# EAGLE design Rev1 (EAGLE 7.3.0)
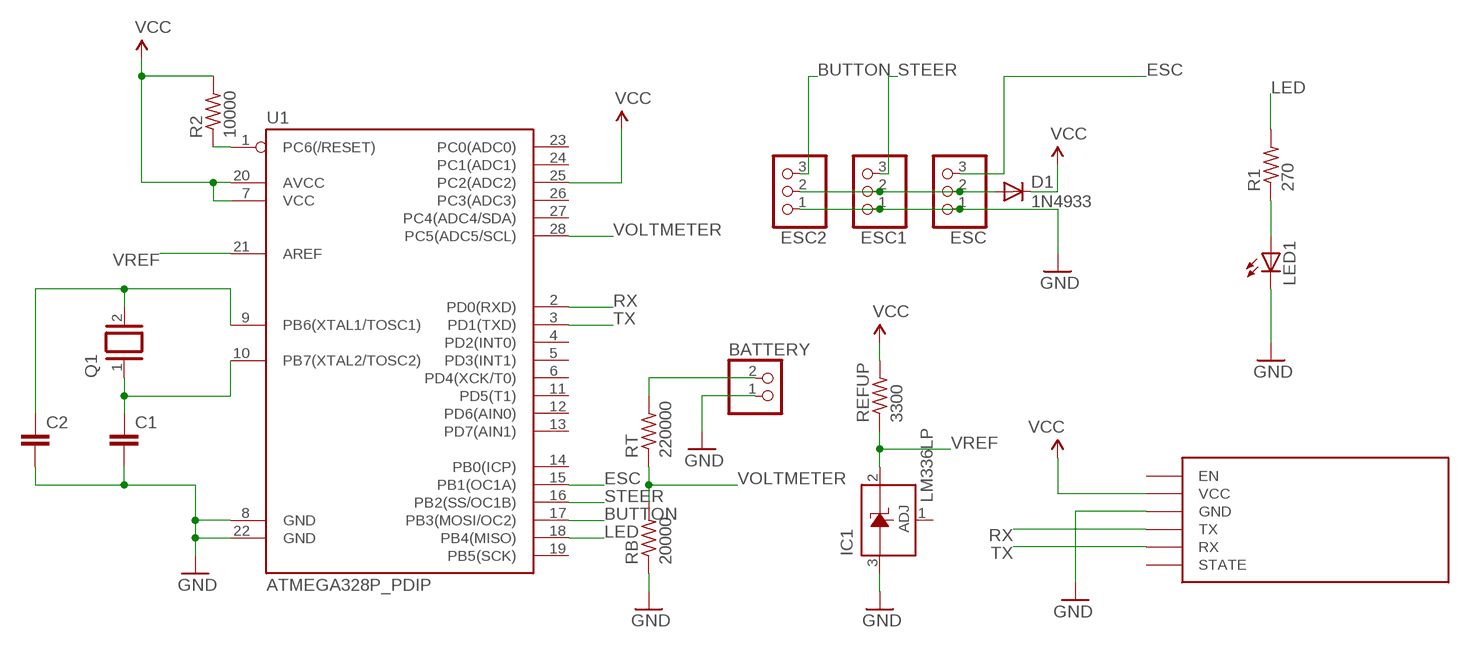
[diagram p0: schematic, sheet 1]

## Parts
BATTERY  JST_2PIN-THM  [JST-PH-2-THM]
C1  C2.5/4  [C2.5-4]
C2  C2.5/4  [C2.5-4]
D1  1N4933  [DO41-10]
ESC  PINHD-1X3  [1X03]
ESC1  PINHD-1X3  [1X03]
ESC2  PINHD-1X3  [1X03]
IC1  LM336LP  [TO92]
LED1  LED5MM  [LED5MM]
Q1  XTAL/S  [QS]
R1  270  R-US_0204/7  [0204/7]
R2  10000  R-US_0207/7  [0207/7]
RB  20000  R-US_0204/7  [0204/7]
REFUP  3300  R-US_0204/7  [0204/7]
RT  220000  R-US_0204/7  [0204/7]
U1  ATMEGA328P_PDIP  [DIL28-3]
U$1  HC06  [HC06]

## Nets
BUTTON: ESC2.3 U1.17(PB3(MOSI/OC2))
ESC: ESC.3 U1.15(PB1(OC1A))
GND: BATTERY.1 C1.2 C2.2 ESC1.1 ESC2.1 ESC.1 IC1.3(A) LED1.K(C) RB.1 U1.8(GND) U1.22(GND) U$1.GND
LED: R1.2 U1.18(PB4(MISO))
N$2: LED1.A R1.1
N$3: C1.1 Q1.1 U1.10(PB7(XTAL2/TOSC2))
N$4: BATTERY.2 RT.2
N$5: C2.1 Q1.2 U1.9(PB6(XTAL1/TOSC1))
N$7: R2.1 U1.1(PC6(/RESET))
N$10: D1.A ESC1.2 ESC2.2 ESC.2
RX: U1.2(PD0(RXD)) U$1.TX
STEER: ESC1.3 U1.16(PB2(SS/OC1B))
TX: U1.3(PD1(TXD)) U$1.RX
VCC: D1.C R2.2 REFUP.2 U1.7(VCC) U1.20(AVCC) U1.25(PC2(ADC2)) U$1.VCC
VOLTMETER: RB.2 RT.1 U1.28(PC5(ADC5/SCL))
VREF: IC1.2(C) REFUP.1 U1.21(AREF)
Unconnected: IC1.1(ADJ) U1.4(PD2(INT0)) U1.5(PD3(INT1)) U1.6(PD4(XCK/T0)) U1.11(PD5(T1)) U1.12(PD6(AIN0)) U1.13(PD7(AIN1)) U1.14(PB0(ICP)) U1.19(PB5(SCK)) U1.23(PC0(ADC0)) U1.24(PC1(ADC1)) U1.26(PC3(ADC3)) U1.27(PC4(ADC4/SDA)) U$1.EN U$1.STATE

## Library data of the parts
BATTERY = adafruit:JST_2PIN: JST 2-Pin Connectors of various flavors
C1 C2 = capacitor-wima:C: CAPACITOR
D1 = diode:1N4933: DIODE
ESC ESC1 ESC2 = pinhead:PINHD-1X3: PIN HEADER
IC1 = VLADLIBRARY:LM336: 2.5-V INTEGRATED REFERENCE CIRCUITS LM236 Source: http://focus.ti.com/lit/ds/symlink/lm336-2.5.pdf
LED1 = adafruit:LED: LED
Q1 = special:XTAL/S: CRYSTAL
R1 RB REFUP RT = adafruit:R-US_: RESISTOR, American symbol
R2 = resistor:R-US_: RESISTOR, American symbol
U1 = SparkFun-DigitalIC:ATMEGA328P_PDIP: uC used in the Arduino 32kb flash, 1k EEPROM, 2k SRAM This is the through-hole version of this chip.
U$1 = ccs:HC06

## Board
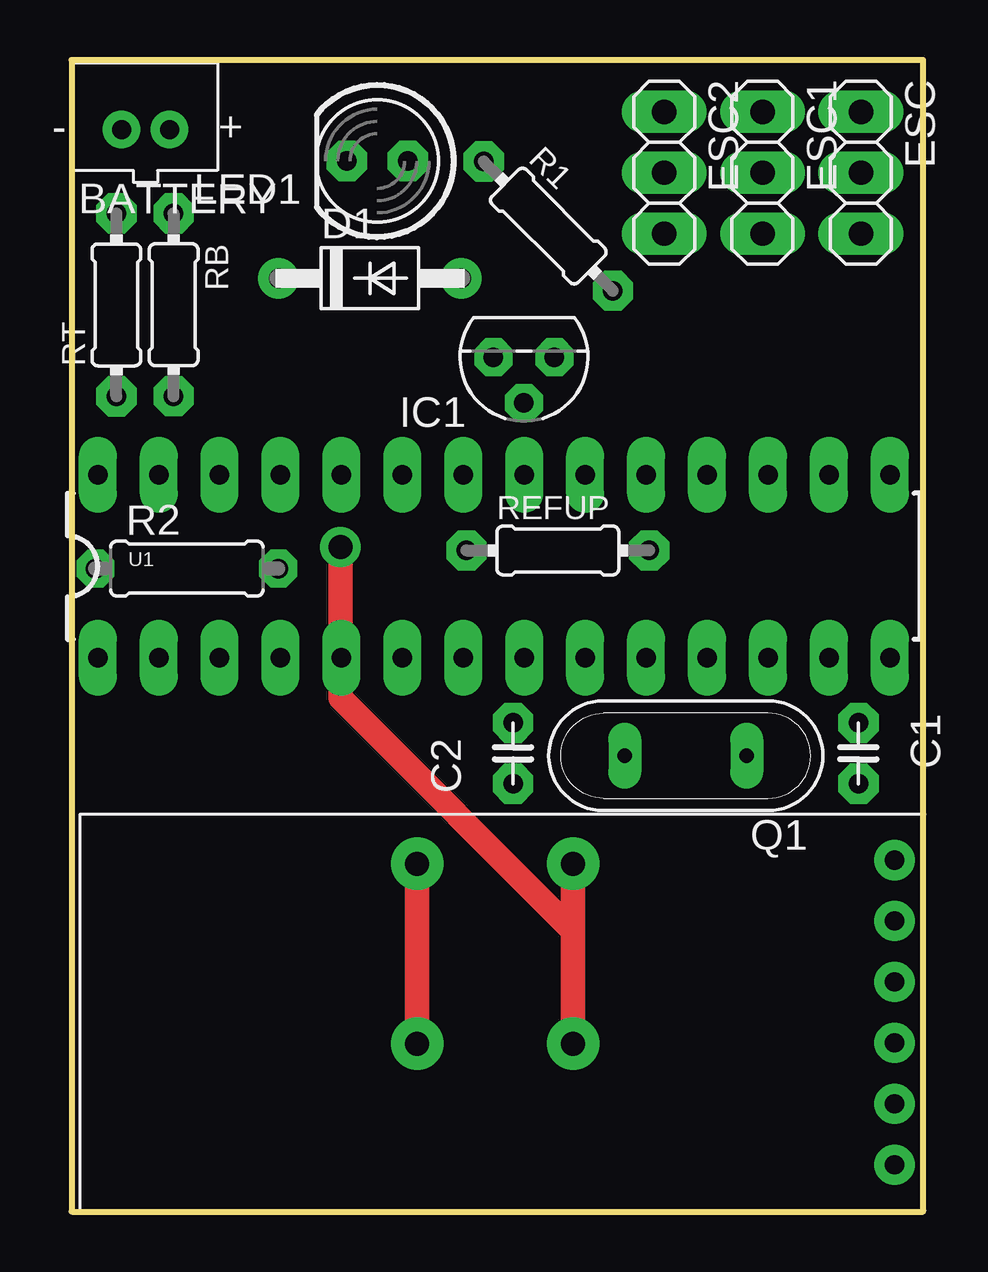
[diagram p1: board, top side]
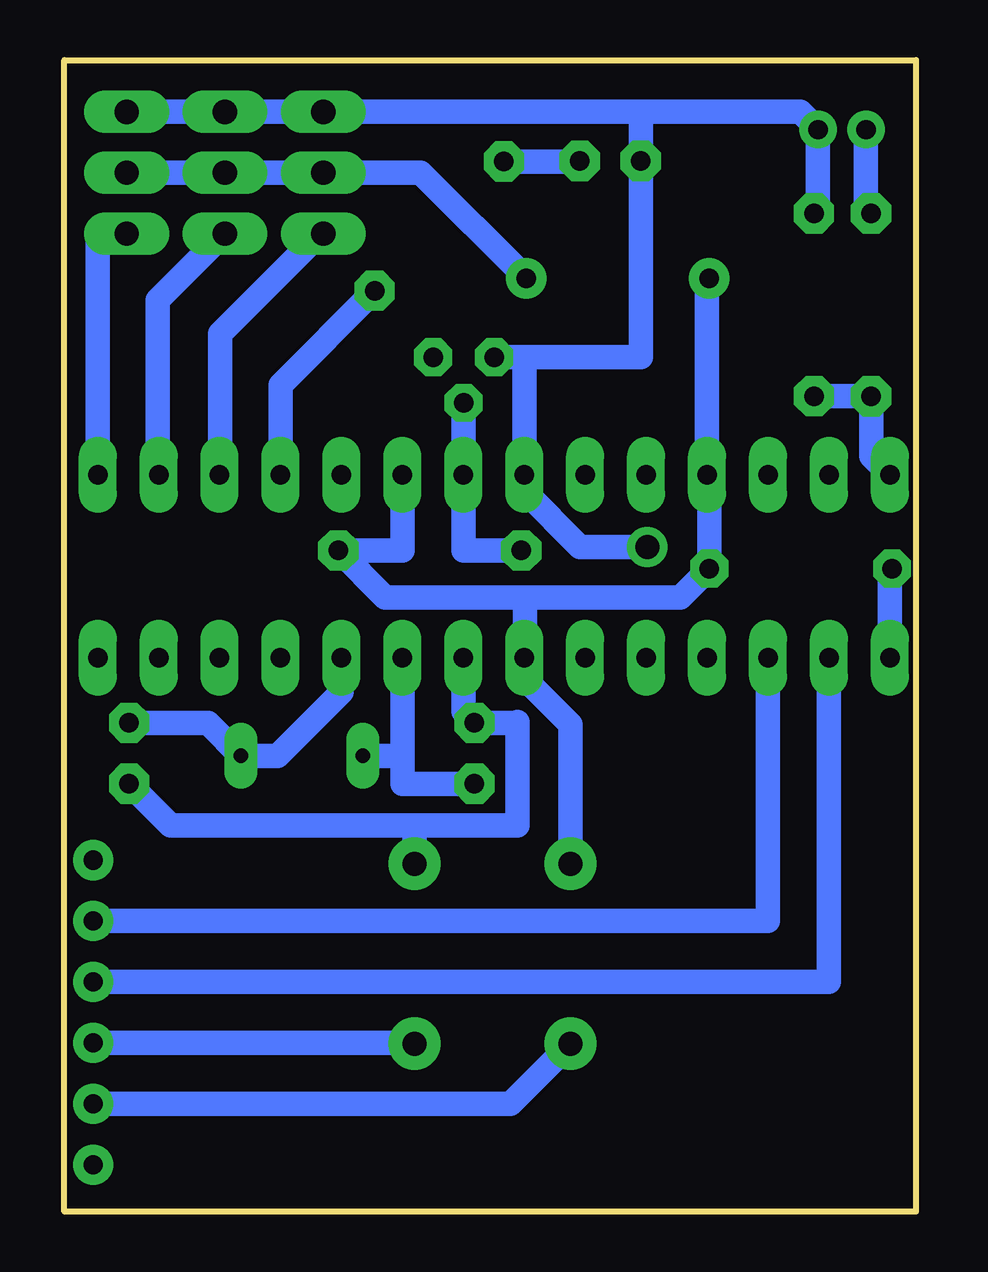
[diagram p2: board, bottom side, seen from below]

Size 35.5 x 48 mm. Coordinates in mm from the lower left corner, seen from the top.
Outline: 0,0 35.5,0 35.5,48 0,48 0,0
Copper layers (1*16): Top 0.035mm / dielectric 1.5mm / Bottom 0.035mm
Design rules "default *": minimum track width 10mil, minimum drill 24mil, track to track 15mil, track to pad 15mil, pad to pad 15mil, via to via 15mil, smd to smd 8mil, copper to edge 40mil, drill to drill 8mil, minimum pad ring 15mil, minimum via ring 8mil, stop-mask expansion 4mil, vias tented up to drill 0mil, thermal gap 10mil

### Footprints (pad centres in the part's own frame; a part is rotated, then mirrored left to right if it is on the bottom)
JST-PH-2-THM = drill 0.8 pad 1.422: 1 1,0; 2 -1,0
C2.5-4 = drill 0.813 pad 1.676 octagon: 1 -1.27,0; 2 1.27,0
DO41-10 = drill 0.8 pad 1.676: A 2.54,0; C -5.08,0
1X03 = drill 1.016 long: 1 -2.54,0; 2 0,0; 3 2.54,0
TO92 = drill 0.813 octagon: 1 -1.27,0; 2 0,1.905; 3 1.27,0
LED5MM = drill 0.813 pad 1.676 octagon: A -1.27,0; K 1.27,0
QS = drill 0.61 long: 1 -2.54,0; 2 2.54,0
0204/7 = drill 0.813 pad 1.676 octagon: 1 -3.81,0; 2 3.81,0
0207/7 = drill 0.813 octagon: 1 -3.81,0; 2 3.81,0
DIL28-3 = drill 0.813 long: 1 -16.51,-3.81; 2 -13.97,-3.81; 3 -11.43,-3.81; 4 -8.89,-3.81; 5 -6.35,-3.81; 6 -3.81,-3.81; 7 -1.27,-3.81; 8 1.27,-3.81; 9 3.81,-3.81; 10 6.35,-3.81; 11 8.89,-3.81; 12 11.43,-3.81; 13 13.97,-3.81; 14 16.51,-3.81; 15 16.51,3.81; 16 13.97,3.81; 17 11.43,3.81; 18 8.89,3.81; 19 6.35,3.81; 20 3.81,3.81; 21 1.27,3.81; 22 -1.27,3.81; 23 -3.81,3.81; 24 -6.35,3.81; 25 -8.89,3.81; 26 -11.43,3.81; 27 -13.97,3.81; 28 -16.51,3.81
HC06 = drill 0.8 pad 1.676: EN -6.35,0; GND -1.27,0; RX 3.81,0; STATE 6.35,0; TX 1.27,0; VCC -3.81,0

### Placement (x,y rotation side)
BATTERY  3.08,45.09 0 top
C1  32.8,19.1 270 top
C2  18.4,19.1 90 top
D1  13.7,38.9 0 top
ESC  32.9,43.3 270 top
ESC1  28.8,43.3 270 top
ESC2  24.7,43.3 270 top
IC1  18.85,35.61 180 top
LED1  12.74,43.79 180 top
Q1  25.6,19 180 top
R1  19.87,41.07 315 top
R2  4.8,26.8 0 top
RB  4.25,37.8 270 top
REFUP  20.27,27.55 0 top
RT  1.86,37.79 90 top
U1  17.6,26.89 0 top
U$1  34.3,8.3 90 top

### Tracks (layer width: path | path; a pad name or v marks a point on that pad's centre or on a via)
BUTTON
  Bottom 1.016: ESC2.3 24.84,40.76 29,36.6 29,30.73 U1.17
ESC
  Bottom 1.016: ESC.3 34.11,40.76 U1.15
GND  (via drill 1 pad 1.68, 1 pad 2.18)
  Top 1.016: v20.9,7 20.9,11.7 | 20.9,11.7 v20.9,14.5 | v11.2,27.7 11.2,21.4 20.9,11.7
  Bottom 1.016: 11.47,45.84 LED1.K 11.47,35.61 IC1.3 16.33,35.61 U1.22 16.33,30.03 14,27.7 v11.2,27.7 | 11.47,45.84 ESC2.1 ESC1.1 ESC.1 | RB.1 4.08,41.78 BATTERY.1 4.83,45.84 11.47,45.84 | U1.8 18.87,20.84 C2.2 16.63,20.37 16.6,20.4 16.6,16.1 20.7,16.1 | C1.2 31.07,16.1 20.7,16.1 | U$1.GND 20.93,7.03 v20.9,7 | v20.9,14.5 20.9,15.9 20.7,16.1
LED
  Bottom 1.016: R1.2 26.49,34.46 U1.18
N$2
  Bottom 1.016: LED1.A 14.01,43.77 R1.1
N$3
  Bottom 1.016: U1.10 23.95,21.65 26.6,19 Q1.1 29.51,20.37 C1.1
N$4
  Bottom 1.016: RT.2 2.08,41.82 BATTERY.2
N$5
  Bottom 1.016: Q1.2 21.41,19 | 21.41,19 U1.9 | C2.1 21.41,17.83 21.41,19
N$7
  Bottom 1.016: R2.1 1.09,26.7 U1.1
N$10
  Bottom 1.016: ESC.2 ESC1.2 ESC2.2 20.64,43.3 D1.A | ESC.2 33.7,43.3 33.6,43.2 33,43.2 | 33,43.2 32.4,43.2 | ESC.2 33,43.2
RX
  Bottom 1.016: U$1.TX 3.63,9.57 U1.2
STEER
  Bottom 1.016: ESC1.3 28.84,40.76 31.6,38 31.6,30.74 U1.16
TX
  Bottom 1.016: U$1.RX 6.17,12.11 U1.3
VCC  (via drill 1 pad 2.18)
  Top 1.016: v14.4,7 v14.4,14.5
  Bottom 1.016: U1.20 21.41,27.55 REFUP.2 22.12,25.6 16.3,25.6 | 16.3,25.6 16.3,23.11 U1.7 16.3,23.06 16.3,22.2 14.4,20.3 v14.4,14.5 | 16.3,25.6 9.81,25.6 R2.2 8.61,30.61 U1.25 8.71,38.81 D1.C | U$1.VCC 16.91,4.49 v14.4,7
VOLTMETER
  Bottom 1.016: U1.28 1.86,31.48 RT.1 1.87,33.99 RB.2
VREF
  Bottom 1.016: IC1.2 18.87,33.69 U1.21 18.87,27.55 REFUP.1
